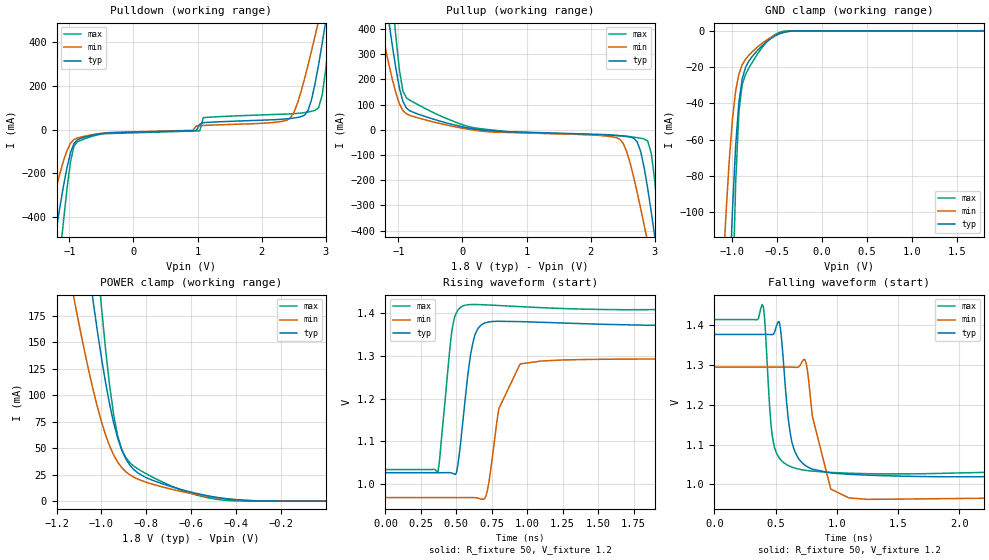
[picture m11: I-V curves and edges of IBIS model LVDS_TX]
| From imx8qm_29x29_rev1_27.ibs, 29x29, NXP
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[Model] LVDS_TX
Model_type   3-state
Polarity   Non-Inverting
Enable   Active-High
Vmeas =   1.2
Cref =   5p
Rref =   50
Vref =   1.2
|   typ   min   max
C_comp  1.9514p   1.9123p   1.9720p
[Temperature Range]   85   125   -40
[Voltage Range]   1.8   1.52   1.98
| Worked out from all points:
|   slope of the pulldown table from 0 to 0.27 V, typ, clamps not added: 132 ohm
|   slope of the pullup table from 0 to 0.27 V, typ, clamps not added: 23.6 ohm
|   GND clamp passes 1 mA (typ) near -0.44 V on its own axis
|   POWER clamp passes 1 mA (typ) near -0.38 V on its own axis
|   falling waveform, R_fixture 50, V_fixture 1.2: 20-80 % time 76.9ps typ, 133ps min, 53.3ps max; typ from 1.38 V to 1.03 V
|   rising waveform, R_fixture 50, V_fixture 1.2: 20-80 % time 72.6ps typ, 133ps min, 65.3ps max; typ from 1.03 V to 1.38 V
[GND_clamp]
|Voltage   I (typ)   I (min)   I (max)
-1.8V     -1.612A    -1.003A    -2.601A
-1.109V   -260.3mA   -136.7mA   -435.1mA
-1.073V   -201.1mA   -102.2mA   -333.3mA
-1.036V   -146.9mA   -72.45mA   -237.4mA
-1V       -99.85mA   -49.02mA   -151.6mA
-963.7mV  -63.22mA   -33.06mA   -84mA
-927.4mV  -39.27mA   -23.8mA    -44.52mA
-891mV    -26.52mA   -18.76mA   -29.65mA
-781.9mV  -14.28mA   -11.66mA   -17.57mA
-527.4mV  -2.88mA    -2.497mA   -2.095mA
-309.2mV  -53.45uA   -70.95uA   -1.209uA
1.8V      36.67nA    192.5uA    5.567nA
[Power_clamp]
|Volatge   I (typ)   I (min)   I (max)
-1.8V     1.693A     1.071A     2.696A
-1.127V   340.2mA    196.7mA    531mA
-1.109V   308mA      176.8mA    477.4mA
-1.036V   187.7mA    104.6mA    273.7mA
-1.018V   160.7mA    89.11mA    227.2mA
-1V       135.4mA    75.08mA    183.6mA
-963.7mV  91.59mA    52.14mA    109.4mA
-927.4mV  59.34mA    36.68mA    61.46mA
-872.8mV  33.76mA    24.71mA    36.12mA
-781.9mV  20.48mA    16.58mA    23.71mA
-527.4mV  5.097mA    4.472mA    3.25mA
-180uV    37.51nA    91.89nA    11.1nA
[Pulldown]
|Volatge   I (typ)   I (min)   I (max)
-1.8V     -1.644A    -1.031A    -2.638A
-1.364V   -763.9mA   -460.1mA   -1.247A
-1.2V     -450mA     -260.2mA   -740.1mA
-1.146V   -351mA     -198.8mA   -576.4mA
-928mV    -63.45mA   -44.97mA   -74.87mA
2.342V    48.7mA     39.51mA    71.34mA
2.615V    59.54mA    175.4mA    76.45mA
2.724V    89.45mA    297.1mA    81.35mA
2.887V    297.8mA    498.9mA    101mA
2.996V    491.6mA    639.6mA    269.8mA
3.105V    699.3mA    783mA      566.7mA
3.595V    1.692A     1.447A     2.106A
[Pullup]
|Volatge   I (typ)   I (min)   I (max)
-1.8V     1.741A     1.108A     2.775A
-1.309V   738.4mA    456mA      1.184A
-1.146V   426.3mA    257.2mA    676.6mA
-1.036V   240.8mA    144.3mA    365.2mA
-981.9mV  165mA      102.1mA    235.1mA
-818.3mV  74.95mA    56.85mA    116.8mA
2.454V    -23.73mA   -37.59mA   -23.66mA
2.727V    -48.82mA   -250.5mA   -31.47mA
2.836V    -152.9mA   -380.5mA   -36.62mA
3V        -424.3mA   -586.8mA   -201.8mA
3.109V    -629.3mA   -728.2mA   -494.9mA
3.599V    -1.612A    -1.381A    -2.021A
[Ramp]
|variable   typ   min   max
dV/dt_r   211m/73p   228m/65p   197m/91p
dV/dt_f   211m/78p   228m/54p   197m/92p
R_load  = 50
[Falling waveform]
R_fixture = 50
V_fixture = 1.2
|time   V (typ)   V (min)   V (max)
0s        1.377V     1.295V     1.414V
400ps     1.377V     1.295V     1.446V
480ps     1.377V     1.295V     1.108V
530ps     1.408V     1.295V     1.066V
640ps     1.098V     1.294V     1.042V
740ps     1.048V     1.313V     1.035V
800ps     1.038V     1.171V     1.033V
950ps     1.028V     988.1mV    1.03V
1.1ns     1.025V     965.6mV    1.028V
3.8ns     1.027V     967.9mV    1.036V
[Rising waveform]
R_fixture = 50
V_fixture = 1.2
|time   V (typ)   V (min)   V (max)
0s        1.026V     967.9mV    1.034V
370ps     1.026V     967.9mV    1.026V
470ps     1.025V     967.9mV    1.363V
500ps     1.025V     967.9mV    1.401V
550ps     1.16V      967.9mV    1.418V
650ps     1.363V     966.8mV    1.42V
710ps     1.378V     973mV      1.419V
800ps     1.381V     1.177V     1.418V
950ps     1.38V      1.281V     1.415V
3.8ns     1.377V     1.295V     1.417V
